(* Logix 5000 AddOnInstructionDefinition export Banner_TL50Select_Param_v4; software revision 33.00; part 2 of 2 *)
(* tags used below, declared in another part *)
   TL50_Pro : Banner_TL50Select_v4;
   Port_Data : Banner_IOL_Port_v4;
   Port : INT;   // Port Number that device is plugged into.
   Local_Control : DINT;
   Command_Being_Processed : BOOL;
   Update_Archive : BOOL;
   Index_Write_Inprocess : DINT;
   Inprocess_Index : DINT;
   SB_W_Index : DINT;
(* Banner_TL50Select_Param_v4, continued *)

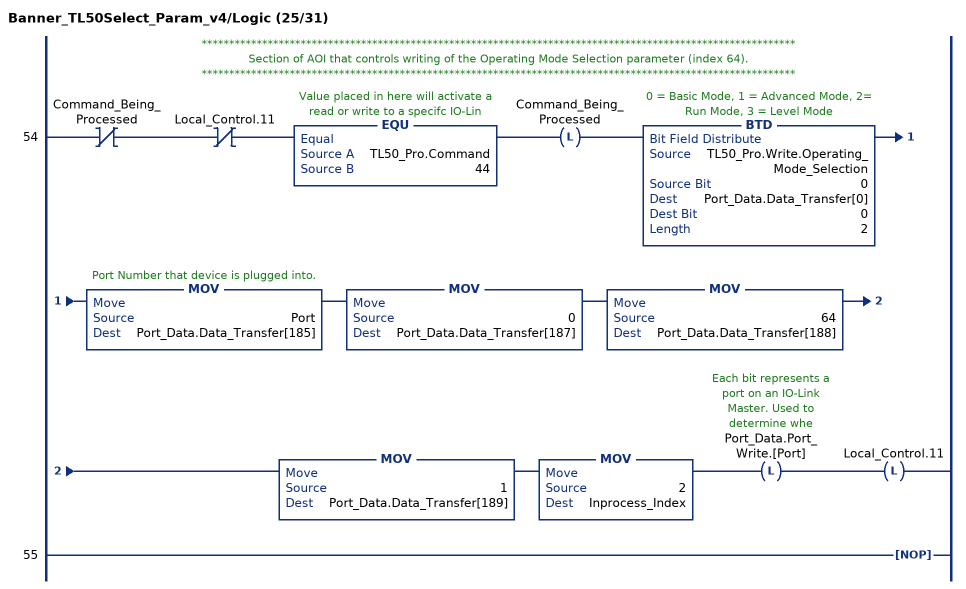
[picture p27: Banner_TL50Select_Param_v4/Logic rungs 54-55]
   // ************************************************************************************************************
   // Section of AOI that controls writing of the Operating Mode Selection parameter (index 64).
   // ************************************************************************************************************
   54: XIO(Command_Being_Processed)XIO(Local_Control.11)EQU(TL50_Pro.Command,44)OTL(Command_Being_Processed)BTD(TL50_Pro.Write.Operating_Mode_Selection,0,Port_Data.Data_Transfer[0],0,2)MOV(Port,Port_Data.Data_Transfer[185])MOV(0,Port_Data.Data_Transfer[187])MOV(64,Port_Data.Data_Transfer[188])MOV(1,Port_Data.Data_Transfer[189])MOV(2,Inprocess_Index)OTL(Port_Data.Port_Write.[Port])OTL(Local_Control.11);
   55: NOP();
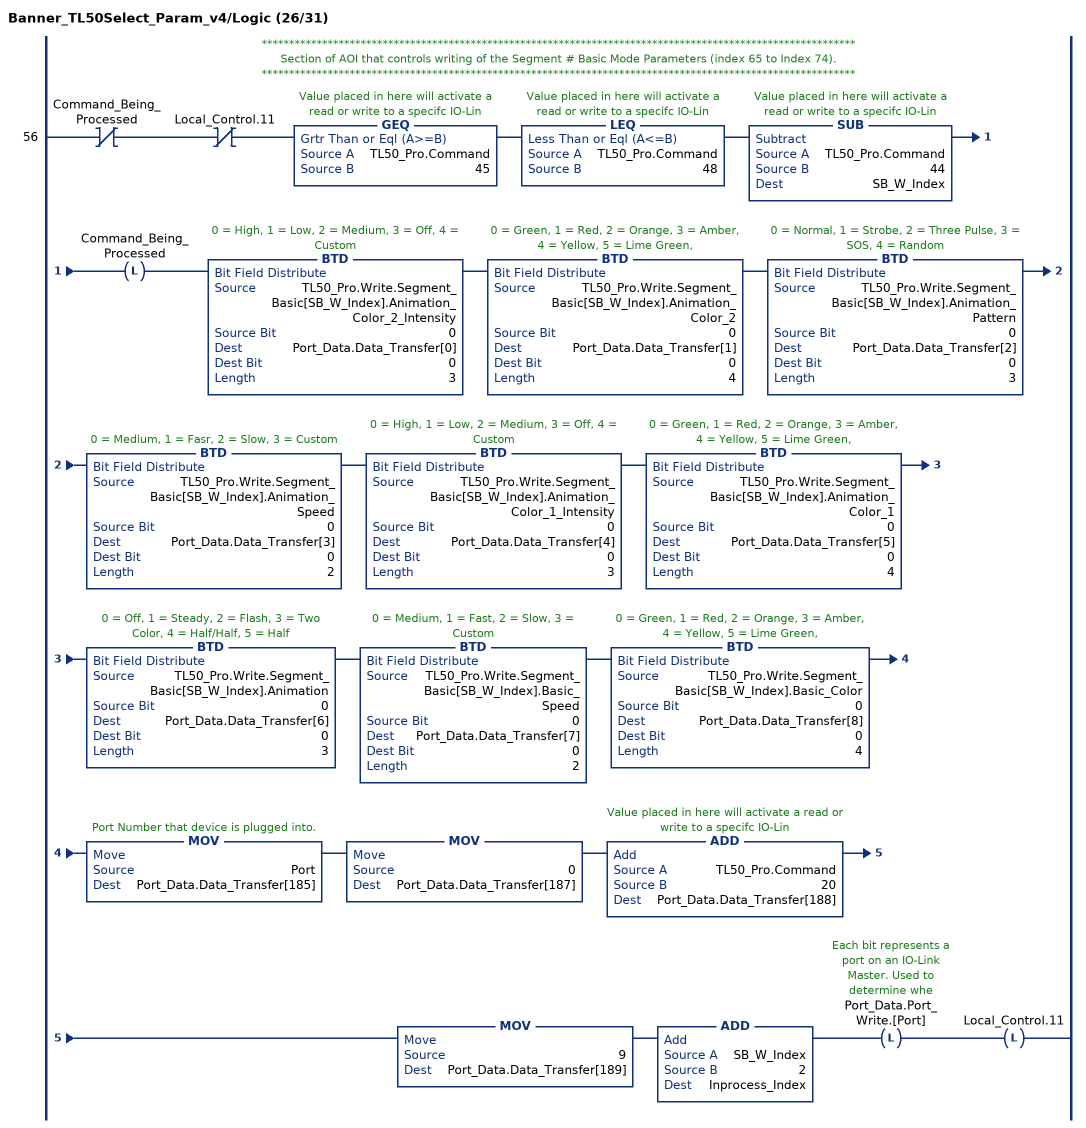
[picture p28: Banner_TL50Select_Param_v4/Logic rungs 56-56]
   // ************************************************************************************************************
   // Section of AOI that controls writing of the Segment # Basic Mode Parameters (index 65 to Index 74).
   // ************************************************************************************************************
   56: XIO(Command_Being_Processed)XIO(Local_Control.11)GEQ(TL50_Pro.Command,45)LEQ(TL50_Pro.Command,48)SUB(TL50_Pro.Command,44,SB_W_Index)OTL(Command_Being_Processed)BTD(TL50_Pro.Write.Segment_Basic[SB_W_Index].Animation_Color_2_Intensity,0,Port_Data.Data_Transfer[0],0,3)BTD(TL50_Pro.Write.Segment_Basic[SB_W_Index].Animation_Color_2,0,Port_Data.Data_Transfer[1],0,4)BTD(TL50_Pro.Write.Segment_Basic[SB_W_Index].Animation_Pattern,0,Port_Data.Data_Transfer[2],0,3)BTD(TL50_Pro.Write.Segment_Basic[SB_W_Index].Animation_Speed,0,Port_Data.Data_Transfer[3],0,2)BTD(TL50_Pro.Write.Segment_Basic[SB_W_Index].Animation_Color_1_Intensity,0,Port_Data.Data_Transfer[4],0,3)BTD(TL50_Pro.Write.Segment_Basic[SB_W_Index].Animation_Color_1,0,Port_Data.Data_Transfer[5],0,4)BTD(TL50_Pro.Write.Segment_Basic[SB_W_Index].Animation,0,Port_Data.Data_Transfer[6],0,3)BTD(TL50_Pro.Write.Segment_Basic[SB_W_Index].Basic_Speed,0,Port_Data.Data_Transfer[7],0,2)BTD(TL50_Pro.Write.Segment_Basic[SB_W_Index].Basic_Color,0,Port_Data.Data_Transfer[8],0,4)MOV(Port,Port_Data.Data_Transfer[185])MOV(0,Port_Data.Data_Transfer[187])ADD(TL50_Pro.Command,20,Port_Data.Data_Transfer[188])MOV(9,Port_Data.Data_Transfer[189])ADD(SB_W_Index,2,Inprocess_Index)OTL(Port_Data.Port_Write.[Port])OTL(Local_Control.11);
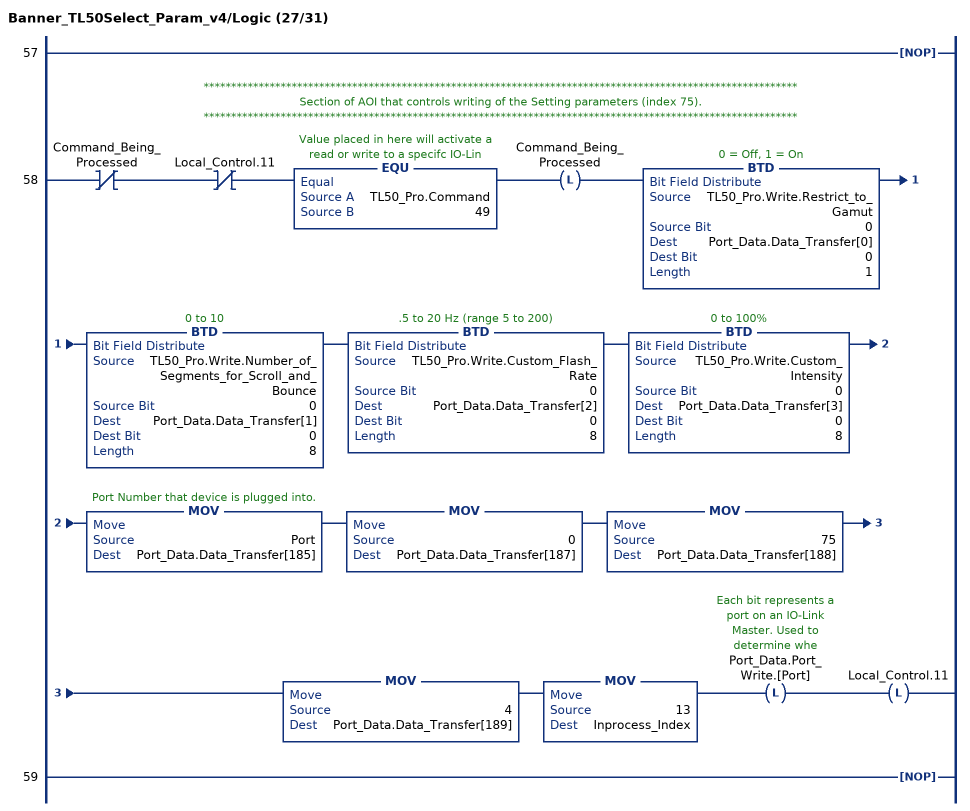
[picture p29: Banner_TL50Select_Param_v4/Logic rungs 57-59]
   57: NOP();
   // ************************************************************************************************************
   // Section of AOI that controls writing of the Setting parameters (index 75).
   // ************************************************************************************************************
   58: XIO(Command_Being_Processed)XIO(Local_Control.11)EQU(TL50_Pro.Command,49)OTL(Command_Being_Processed)BTD(TL50_Pro.Write.Restrict_to_Gamut,0,Port_Data.Data_Transfer[0],0,1)BTD(TL50_Pro.Write.Number_of_Segments_for_Scroll_and_Bounce,0,Port_Data.Data_Transfer[1],0,8)BTD(TL50_Pro.Write.Custom_Flash_Rate,0,Port_Data.Data_Transfer[2],0,8)BTD(TL50_Pro.Write.Custom_Intensity,0,Port_Data.Data_Transfer[3],0,8)MOV(Port,Port_Data.Data_Transfer[185])MOV(0,Port_Data.Data_Transfer[187])MOV(75,Port_Data.Data_Transfer[188])MOV(4,Port_Data.Data_Transfer[189])MOV(13,Inprocess_Index)OTL(Port_Data.Port_Write.[Port])OTL(Local_Control.11);
   59: NOP();
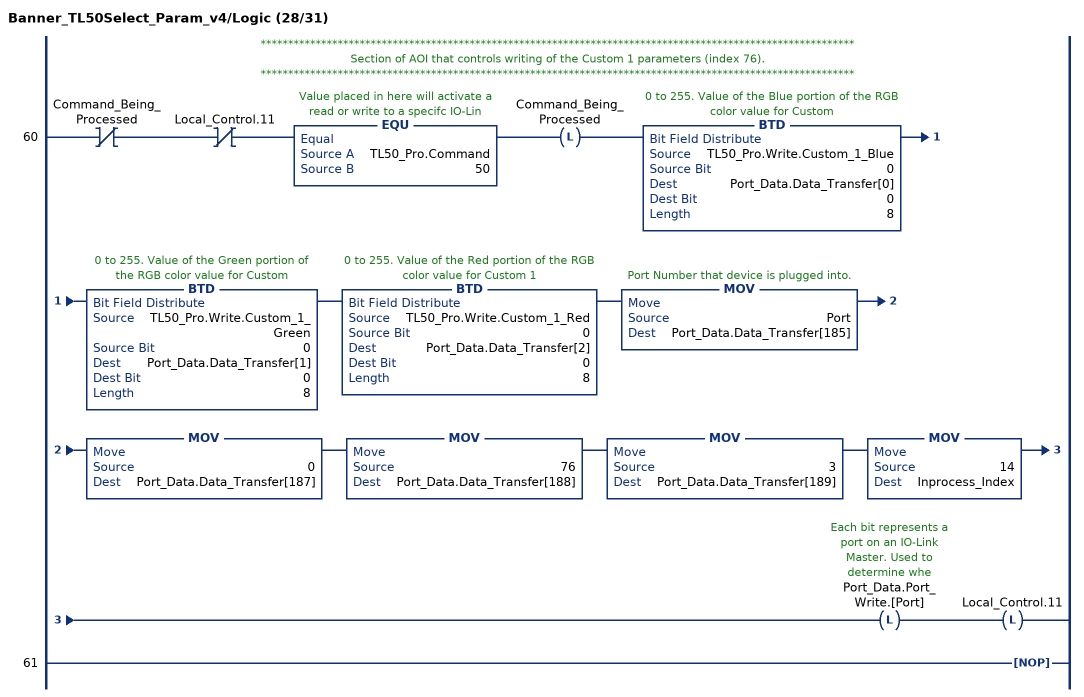
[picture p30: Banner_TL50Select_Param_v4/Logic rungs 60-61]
   // ************************************************************************************************************
   // Section of AOI that controls writing of the Custom 1 parameters (index 76).
   // ************************************************************************************************************
   60: XIO(Command_Being_Processed)XIO(Local_Control.11)EQU(TL50_Pro.Command,50)OTL(Command_Being_Processed)BTD(TL50_Pro.Write.Custom_1_Blue,0,Port_Data.Data_Transfer[0],0,8)BTD(TL50_Pro.Write.Custom_1_Green,0,Port_Data.Data_Transfer[1],0,8)BTD(TL50_Pro.Write.Custom_1_Red,0,Port_Data.Data_Transfer[2],0,8)MOV(Port,Port_Data.Data_Transfer[185])MOV(0,Port_Data.Data_Transfer[187])MOV(76,Port_Data.Data_Transfer[188])MOV(3,Port_Data.Data_Transfer[189])MOV(14,Inprocess_Index)OTL(Port_Data.Port_Write.[Port])OTL(Local_Control.11);
   61: NOP();
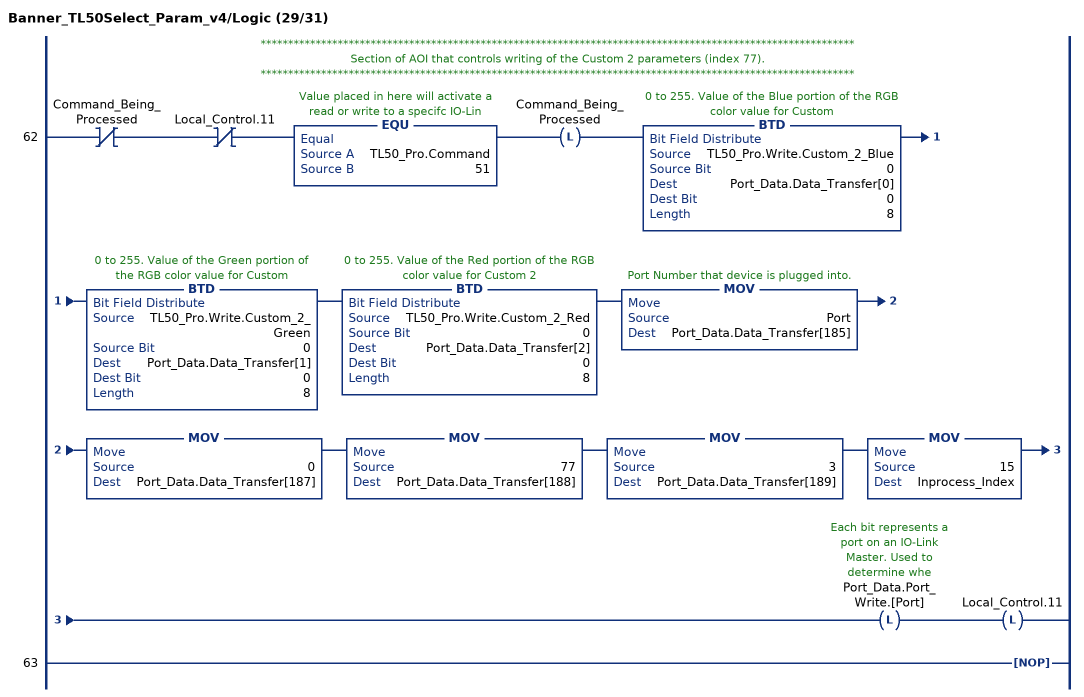
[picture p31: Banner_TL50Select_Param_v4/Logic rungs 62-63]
   // ************************************************************************************************************
   // Section of AOI that controls writing of the Custom 2 parameters (index 77).
   // ************************************************************************************************************
   62: XIO(Command_Being_Processed)XIO(Local_Control.11)EQU(TL50_Pro.Command,51)OTL(Command_Being_Processed)BTD(TL50_Pro.Write.Custom_2_Blue,0,Port_Data.Data_Transfer[0],0,8)BTD(TL50_Pro.Write.Custom_2_Green,0,Port_Data.Data_Transfer[1],0,8)BTD(TL50_Pro.Write.Custom_2_Red,0,Port_Data.Data_Transfer[2],0,8)MOV(Port,Port_Data.Data_Transfer[185])MOV(0,Port_Data.Data_Transfer[187])MOV(77,Port_Data.Data_Transfer[188])MOV(3,Port_Data.Data_Transfer[189])MOV(15,Inprocess_Index)OTL(Port_Data.Port_Write.[Port])OTL(Local_Control.11);
   63: NOP();
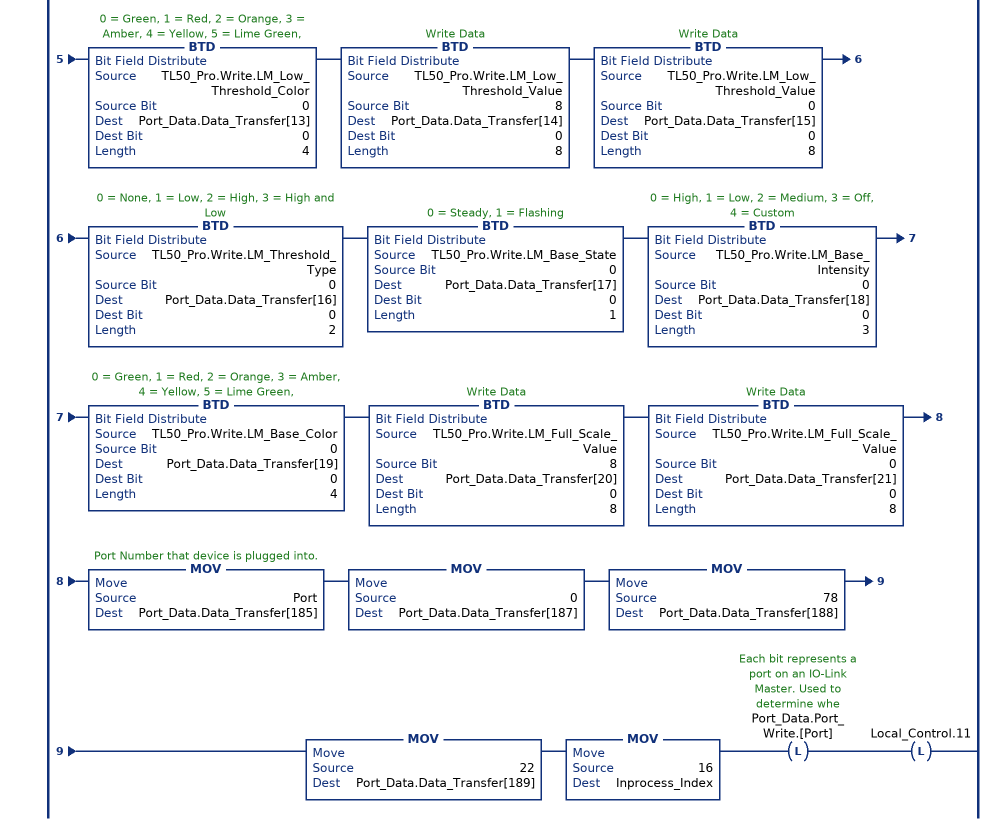
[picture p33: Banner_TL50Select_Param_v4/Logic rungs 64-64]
   // ************************************************************************************************************
   // Section of AOI that controls writing of the LeveL Mode Configuration parameters (index 78).
   // ************************************************************************************************************
   64: XIO(Command_Being_Processed)XIO(Local_Control.11)EQU(TL50_Pro.Command,52)OTL(Command_Being_Processed)BTD(TL50_Pro.Write.LM_Orientation,0,Port_Data.Data_Transfer[0],0,1)BTD(TL50_Pro.Write.LM_Background_Intensity,0,Port_Data.Data_Transfer[1],0,3)BTD(TL50_Pro.Write.LM_Background_Color,0,Port_Data.Data_Transfer[2],0,4)BTD(TL50_Pro.Write.LM_Subsegment_Style,0,Port_Data.Data_Transfer[3],0,2)BTD(TL50_Pro.Write.LM_Dominance,0,Port_Data.Data_Transfer[4],0,1)BTD(TL50_Pro.Write.LM_Flash_Rate,0,Port_Data.Data_Transfer[5],0,2)BTD(TL50_Pro.Write.LM_High_Threshold_State,0,Port_Data.Data_Transfer[6],0,1)BTD(TL50_Pro.Write.LM_High_Threshold_Intensity,0,Port_Data.Data_Transfer[7],0,3)BTD(TL50_Pro.Write.LM_High_Threshold_Color,0,Port_Data.Data_Transfer[8],0,4)BTD(TL50_Pro.Write.LM_High_Threshold_Value,8,Port_Data.Data_Transfer[9],0,8)BTD(TL50_Pro.Write.LM_High_Threshold_Value,0,Port_Data.Data_Transfer[10],0,8)BTD(TL50_Pro.Write.LM_Low_Threshold_State,0,Port_Data.Data_Transfer[11],0,1)BTD(TL50_Pro.Write.LM_Low_Threshold_Intensity,0,Port_Data.Data_Transfer[12],0,3)BTD(TL50_Pro.Write.LM_Low_Threshold_Color,0,Port_Data.Data_Transfer[13],0,4)BTD(TL50_Pro.Write.LM_Low_Threshold_Value,8,Port_Data.Data_Transfer[14],0,8)BTD(TL50_Pro.Write.LM_Low_Threshold_Value,0,Port_Data.Data_Transfer[15],0,8)BTD(TL50_Pro.Write.LM_Threshold_Type,0,Port_Data.Data_Transfer[16],0,2)BTD(TL50_Pro.Write.LM_Base_State,0,Port_Data.Data_Transfer[17],0,1)BTD(TL50_Pro.Write.LM_Base_Intensity,0,Port_Data.Data_Transfer[18],0,3)BTD(TL50_Pro.Write.LM_Base_Color,0,Port_Data.Data_Transfer[19],0,4)BTD(TL50_Pro.Write.LM_Full_Scale_Value,8,Port_Data.Data_Transfer[20],0,8)BTD(TL50_Pro.Write.LM_Full_Scale_Value,0,Port_Data.Data_Transfer[21],0,8)MOV(Port,Port_Data.Data_Transfer[185])MOV(0,Port_Data.Data_Transfer[187])MOV(78,Port_Data.Data_Transfer[188])MOV(22,Port_Data.Data_Transfer[189])MOV(16,Inprocess_Index)OTL(Port_Data.Port_Write.[Port])OTL(Local_Control.11);
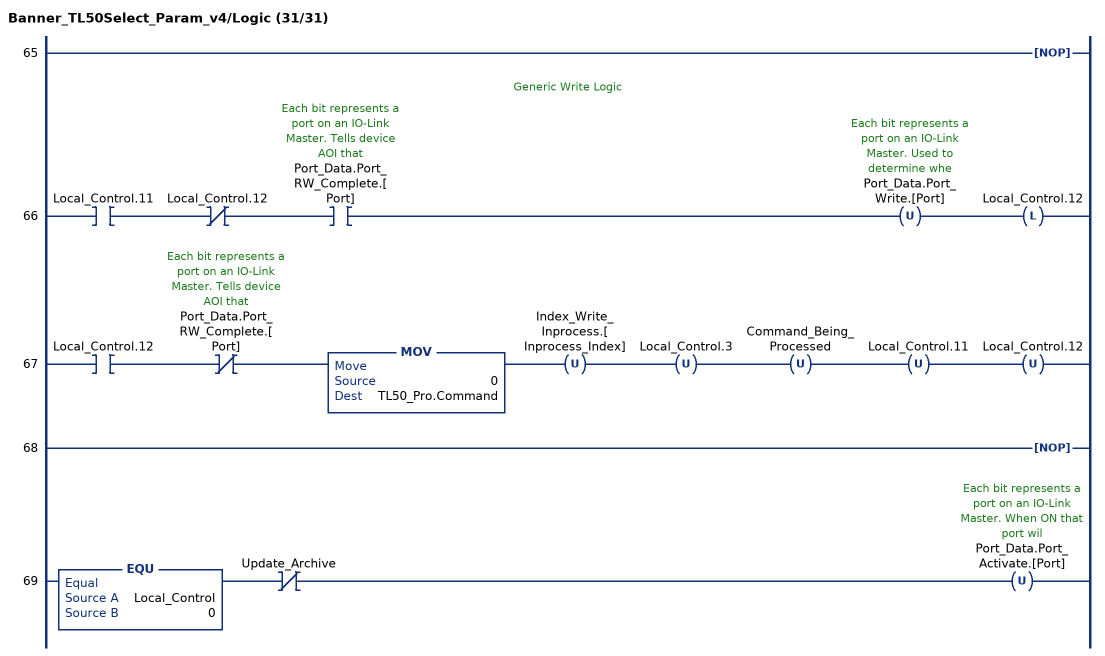
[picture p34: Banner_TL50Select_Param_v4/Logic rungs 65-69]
   65: NOP();
   // Generic Write Logic
   66: XIC(Local_Control.11)XIO(Local_Control.12)XIC(Port_Data.Port_RW_Complete.[Port])OTU(Port_Data.Port_Write.[Port])OTL(Local_Control.12);
   67: XIC(Local_Control.12)XIO(Port_Data.Port_RW_Complete.[Port])MOV(0,TL50_Pro.Command)OTU(Index_Write_Inprocess.[Inprocess_Index])OTU(Local_Control.3)OTU(Command_Being_Processed)OTU(Local_Control.11)OTU(Local_Control.12);
   68: NOP();
   69: EQU(Local_Control,0)XIO(Update_Archive)OTU(Port_Data.Port_Activate.[Port]);
END_ROUTINE
END_ADD_ON_INSTRUCTION
